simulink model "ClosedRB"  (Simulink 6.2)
settings: Solver=ode45  StartTime=0.0  StopTime=5  MaxStep=0.05  RelTol=1e-3
undefined symbols (not defined in the file or in its folder): Ar, Br, Cr, Dr

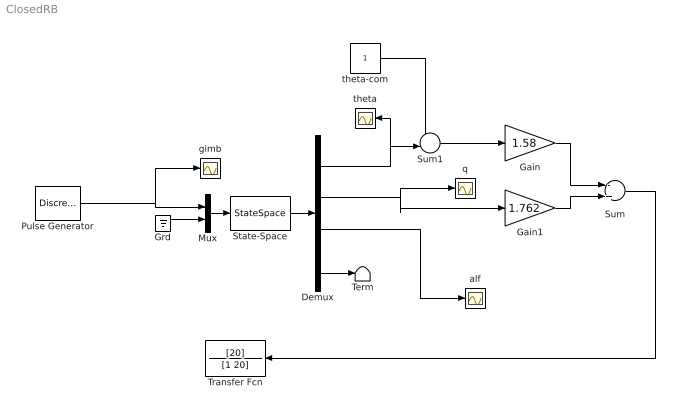
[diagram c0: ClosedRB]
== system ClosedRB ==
  Demux : Demux
  Gain : Gain  Gain=1.58
  Gain1 : Gain  Gain=1.762
  Grd : Ground
  Mux : Mux  Inputs=2
  Pulse Generator : DiscretePulseGenerator  PulseType=Time based  Period=10
  State-Space : StateSpace  A=Ar  B=Br  C=Cr  D=Dr
  Sum : Sum  Inputs=-+
  Sum1 : Sum  Inputs=+-|
  Term : Terminator
  Transfer Fcn : TransferFcn  Orientation=left  Numerator=[20]  Denominator=[1 20]
  alf : Scope
  gimb : Scope
  q : Scope
  theta : Scope
  theta-com : Constant
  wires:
  Mux/1 -> State-Space/1
  Demux/4 -> Term/1
  Grd/1 -> Mux/2
  Gain1/1 -> Sum/2
  Gain/1 -> Sum/1
  Sum/1 -> Transfer Fcn/1
  Sum1/1 -> Gain/1
  Demux/1 -> Sum1/2, theta/1
  theta-com/1 -> Sum1/1
  State-Space/1 -> Demux/1
  Demux/2 -> Gain1/1, q/1
  Demux/3 -> alf/1
  Pulse Generator/1 -> Mux/1, gimb/1
